PROGRAM MAIN
VAR
	x: UINT :=0;
	a AT %Q* :UINT := 1;
	output AT %Q* :UINT;
	in_main AT %I* :BYTE :=0;
	bMainOut5 AT %Q* :REAL := 0;
	mark : BOOL :=FALSE;
	RELAISOUT AT %Q* :BOOL :=TRUE;
	
	RELAY_IN_B AT %I* :REAL:= 0.0;
	
	RELAY AT %Q* :REAL;
	
	
END_VAR

x := x+ 1;
Iridium.x[0] :=1;
IF bMainOut5 < 10 THEN
	mark :=TRUE;
END_IF
IF bMainOut5 <> 5 THEN
	mark :=FALSE;
END_IF

END_PROGRAM
